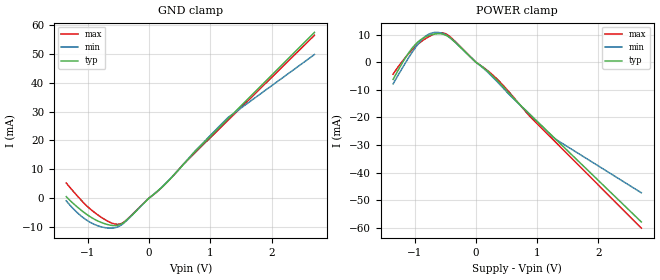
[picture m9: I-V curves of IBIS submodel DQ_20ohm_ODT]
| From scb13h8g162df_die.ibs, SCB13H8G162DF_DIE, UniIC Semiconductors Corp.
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|   Submodel DQ_20ohm_ODT
[Submodel] DQ_20ohm_ODT
Submodel_type Dynamic_clamp
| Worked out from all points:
|   GND clamp passes 1 mA (typ) near -0.05 V on its own axis
|   POWER clamp passes 1 mA (typ) near -0.05 V on its own axis
[GND_clamp]
|Voltage   I(typ)   I(min)   I(max)
-1.35V    480.8uA    -971.8uA   5.219mA
-1.097V   -4.389mA   -6.428mA   -953.7uA
-872mV    -7.575mA   -9.334mA   -5.281mA
-591mV    -9.552mA   -10.43mA   -8.82mA
-506mV    -9.456mA   -9.991mA   -9.129mA
-422mV    -8.652mA   -8.905mA   -8.533mA
-100nV    1.004nA    10.15nA    -1.612nA
253mV     4.636mA    4.686mA    4.582mA
562mV     11.66mA    11.74mA    11.78mA
759mV     16.19mA    16.49mA    15.9mA
1.294V    27.58mA    28.03mA    27.1mA
2.7V      57.55mA    49.85mA    56.55mA
[POWER_clamp]
|Voltage   I(typ)   I(min)   I(max)
-1.35V    -6.238mA   -7.864mA   -4.348mA
-1.069V   4.228mA    2.604mA    3.82mA
-956mV    7.109mA    6.2mA      6.28mA
-844mV    8.931mA    8.99mA     8.207mA
-675mV    10.21mA    10.76mA    10.2mA
-562mV    10.24mA    10.56mA    10.65mA
-478mV    9.621mA    9.749mA    10.12mA
100nV     -190nA     -185.8nA   -197.9nA
338mV     -6.409mA   -6.81mA    -5.913mA
872mV     -18.68mA   -18.76mA   -19.4mA
1.294V    -27.72mA   -27.77mA   -28.79mA
2.7V      -57.84mA   -47.28mA   -60.08mA
